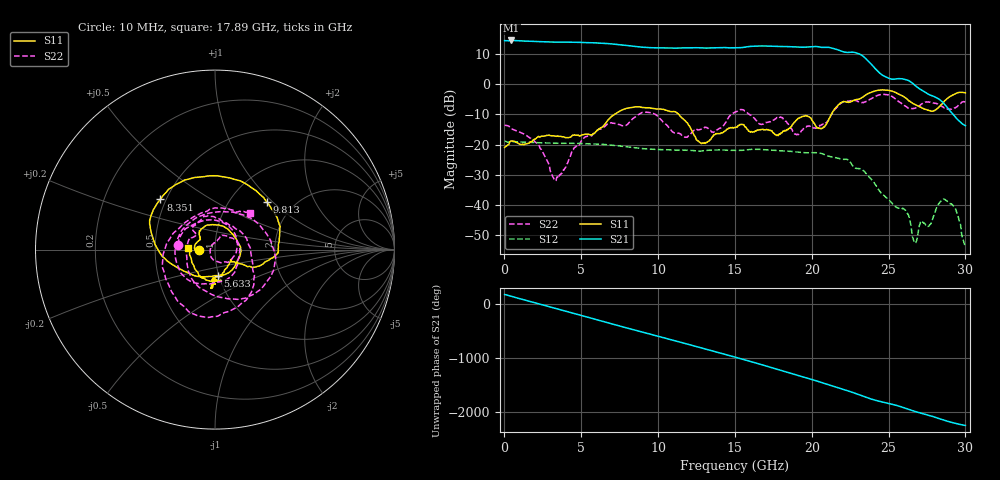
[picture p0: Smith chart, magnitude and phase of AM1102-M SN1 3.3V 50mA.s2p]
!Agilent Technologies,E8364B,MY43040894,A.07.50.67
!Agilent E8364B: A.07.50.67
!Date: Monday, May 24, 2021 14:24:29
!Correction: S11(Full 2 Port(1,2))
!S21(Full 2 Port(1,2))
!S12(Full 2 Port(1,2))
!S22(Full 2 Port(1,2))
!S2P File: Measurements: S11, S21, S12, S22:
# Hz S  dB  R 50
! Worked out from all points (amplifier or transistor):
!   1601 points, 10 MHz to 30 GHz, reference 50 ohm
!   highest |S21| = 14.5 dB at 441.1 MHz (marker M1)
!   |S21| within 3 dB of that: start of sweep to 21.64 GHz
!   unconditionally stable (mu >= 1): start of sweep to end of sweep
!   at 4.996 GHz: K = 1.21, MAG = 13.9 dB, |S12| = -19.6 dB
!   at 15.01 GHz: K = 1.52, MAG = 12.7 dB, |S12| = -21.9 dB
!   at 30 GHz: K = 412.63, MAG = -9.2 dB, |S12| = -53.6 dB
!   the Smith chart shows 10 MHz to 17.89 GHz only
!   S11 on the Smith chart (normalised r, x): 10 MHz: 0.84, -0.01; 5.633 GHz: 0.99, -0.29; 8.351 GHz: 0.47, +0.31; 9.813 GHz: 1.47, +0.92; 17.89 GHz: 0.74, +0.02
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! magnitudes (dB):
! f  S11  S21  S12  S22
! 10 MHz  -20.9  14.4  -18.8  -13.6
! 441.1 MHz  -18.8  14.5  -19.0  -14.7
! 2.128 GHz  -17.6  14.1  -19.3  -19.6
! 3.271 GHz  -17.2  13.9  -19.5  -31.6
! 5.015 GHz  -16.8  13.8  -19.6  -18.7
! 5.633 GHz  -16.7  13.7  -19.7  -17.1
! 8.351 GHz  -7.7  12.6  -20.9  -11.4
! 9.813 GHz  -8.1  12.0  -21.6  -10.0
! 10.02 GHz  -8.2  12.0  -21.6  -10.8
! 11.72 GHz  -11.9  12.0  -21.8  -17.5
! 12.81 GHz  -19.6  12.0  -22.1  -14.9
! 15.01 GHz  -14.3  12.0  -21.9  -9.2
! 17.89 GHz  -16.4  12.5  -22.0  -10.9
! 20.01 GHz  -11.9  12.4  -22.6  -14.3
! 20.7 GHz  -14.6  12.2  -23.0  -13.4
! 22.35 GHz  -6.0  10.5  -25.0  -5.6
! 25.01 GHz  -2.1  2.0  -38.3  -3.6
! 26.18 GHz  -4.8  1.4  -42.3  -7.5
! 26.72 GHz  -6.7  -0.4  -52.6  -7.9
! 28.71 GHz  -5.3  -7.0  -38.3  -8.0
! 29.38 GHz  -3.0  -11.1  -41.6  -7.6
! 30 GHz  -2.8  -13.7  -53.6  -5.9
